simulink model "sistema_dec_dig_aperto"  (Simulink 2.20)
settings: Solver=VariableStepDiscrete  StartTime=0.0  StopTime=10.0  RelTol=1e-3  AbsTol=1e-6

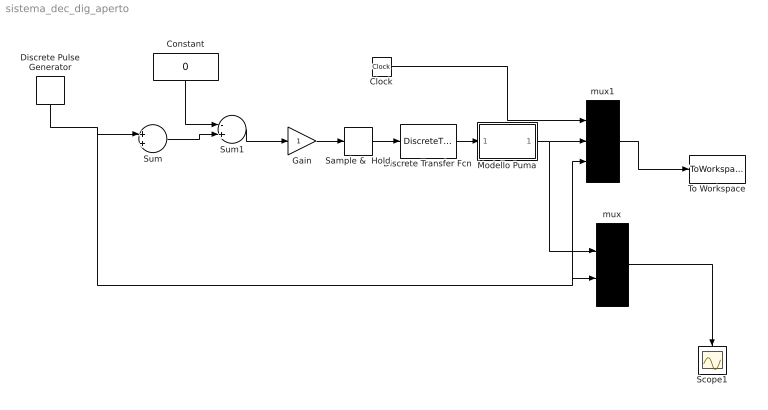
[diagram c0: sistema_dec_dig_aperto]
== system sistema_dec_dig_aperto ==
  Clock : Clock
  Constant : Constant  Orientation=down  Value=0
  Discrete Transfer Fcn : DiscreteTransferFcn  Numerator=1  Denominator=[1 0 0 0 0 0 0 0 0]  SampleTime=.032
  Discrete Pulse Generator : DiscretePulseGenerator  Orientation=down  Amplitude=1  Period=100  PulseWidth=26  PhaseDelay=4  SampleTime=.1
  Gain : Gain  Gain=1
  Modello Puma : Subsystem  Description=Modello Puma
  Sample &  Hold : ZeroOrderHold  SampleTime=.260
  Scope1 : Scope
  Sum : Sum  Inputs=++
  Sum1 : Sum  Inputs=-+
  To Workspace : ToWorkspace  VariableName=sim  SampleTime=-1
  mux : Mux  Inputs=2
  mux1 : Mux  Inputs=3
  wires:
  Sum/1 -> Sum1/2
  Constant/1 -> Sum1/1
  Gain/1 -> Sample &  Hold/1
  Discrete Transfer Fcn/1 -> Modello Puma/1(In1)
  Sample &  Hold/1 -> Discrete Transfer Fcn/1
  Sum1/1 -> Gain/1
  Clock/1 -> mux1/1
  Discrete Pulse Generator/1 -> Sum/1, mux1/3, mux/2
  mux1/1 -> To Workspace/1
  mux/1 -> Scope1/1
  Modello Puma/1(Out1) -> mux1/2, mux/1

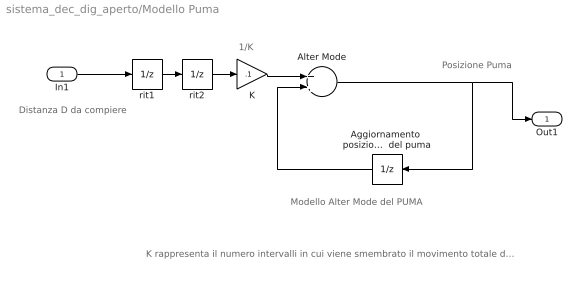
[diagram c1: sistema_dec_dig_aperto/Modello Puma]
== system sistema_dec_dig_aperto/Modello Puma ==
  note: Posizione Puma
  note: Modello Alter Mode del PUMA
  note: 1/K
  note: K rappresenta il numero intervalli in cui viene smembrato il movimento totale da compiere, dopo K time-slice (del PUMA) si ottiene che si e' compiuto proprio la distanza D trasmessa.
  note: Distanza D da compiere
  In1 : Inport  Port=1  PortWidth=-1  SampleTime=-1
  Aggiornamento  posizione   Il sample-time di questo blocco rappresenta la TIME-SLICE  del puma : UnitDelay  Orientation=left  X0=0  SampleTime=.032
  Alter Mode : Sum  Inputs=++
  K : Gain  Gain=.1
  rit1 : UnitDelay  X0=0  SampleTime=.032
  rit2 : UnitDelay  X0=0  SampleTime=.032
  Out1 : Outport  Port=1
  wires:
  K/1 -> Alter Mode/1
  Aggiornamento  posizione   Il sample-time di questo blocco rappresenta la TIME-SLICE  del puma/1 -> Alter Mode/2
  Alter Mode/1 -> Out1/1, Aggiornamento  posizione   Il sample-time di questo blocco rappresenta la TIME-SLICE  del puma/1
  rit2/1 -> K/1
  rit1/1 -> rit2/1
  In1/1 -> rit1/1
